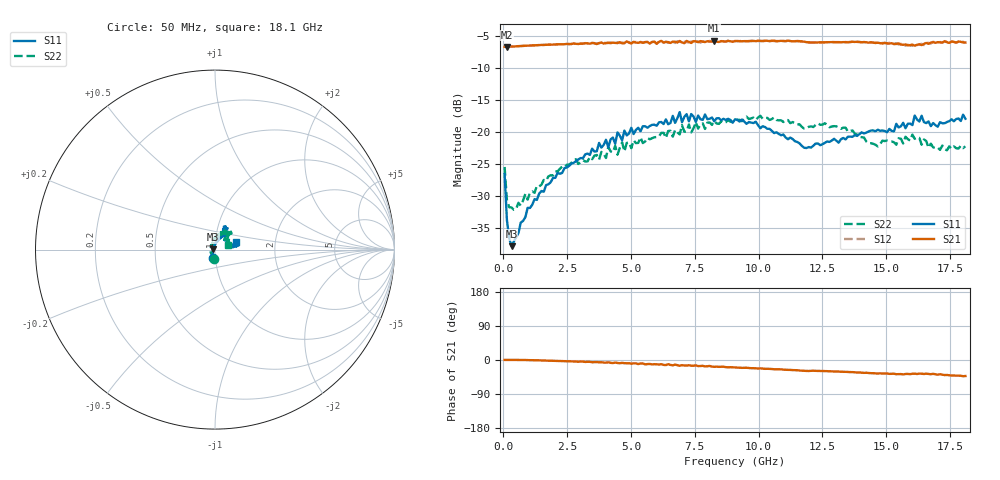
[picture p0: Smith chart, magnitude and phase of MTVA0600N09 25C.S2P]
! Network Analyzer HP8720D.06.14 Serial No. US36140669
!  7 Jul 2005  06:27:09
! Frequency  S11  S21  S12  S22
# HZ  S  DB R 50
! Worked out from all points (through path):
!   201 points, 50 MHz to 18.1 GHz, reference 50 ohm
!   highest |S21| = -5.68 dB at 8.263 GHz (marker M1); lowest = -6.7 dB at 140.2 MHz (marker M2)
!   group delay of S21, straight-line fit = 6.97 ps
!   lowest |S11| = -37.9 dB at 320.8 MHz (marker M3), VSWR 1.03, Z = 48.7 + j0.0733 ohm
!   |S11| at or under -10 dB: start of sweep to end of sweep
!   |S22| runs from -32.2 to -17.5 dB; largest |S21 - S12| = 0.019
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5e7  -26.57 -102.2  -6.65 0.3  -6.68 0.4  -25.48 -94.9
1.4025e8  -33.81 -127.1  -6.69 0.3  -6.68 0.3  -30.67 -144.8
3.2075e8  -37.89 176.6  -6.60 0.5  -6.63 0.5  -31.83 177.1
1.22325e9  -30.52 95.2  -6.43 -0.6  -6.45 -0.6  -29.54 115.1
3.1185e9  -24.10 70.9  -6.16 -4.2  -6.20 -4.5  -24.40 93.6
4.382e9  -21.86 64.8  -6.05 -6.7  -6.05 -7.9  -22.16 85.1
4.47225e9  -20.07 61.2  -6.08 -7.8  -5.97 -7.1  -23.56 87.4
4.65275e9  -21.30 61.3  -6.11 -7.5  -5.98 -8.5  -21.61 86.3
4.743e9  -19.79 64.6  -6.10 -8.4  -6.04 -7.8  -23.05 81.9
6.09675e9  -18.50 63.1  -5.89 -12.0  -5.81 -11.9  -20.72 71.2
6.7285e9  -18.57 67.7  -5.87 -12.1  -6.06 -12.6  -19.69 63.7
6.909e9  -16.89 66.0  -5.75 -15.1  -5.83 -13.8  -20.38 61.6
6.99925e9  -18.48 65.4  -5.97 -13.6  -6.09 -14.9  -18.93 63.2
7.36025e9  -17.19 59.2  -6.05 -15.2  -5.83 -14.6  -20.07 66.2
8.26275e9  -18.34 64.4  -5.68 -18.0  -5.83 -18.4  -18.30 52.9
9.075e9  -18.02 63.3  -5.77 -19.6  -5.74 -19.6  -18.16 50.9
1.21435e10  -22.16 44.6  -5.99 -28.4  -5.95 -28.6  -19.23 52.8
1.512175e10  -19.52 9.6  -6.16 -36.6  -6.03 -36.4  -21.47 41.8
1.602425e10  -18.92 14.4  -6.32 -36.3  -6.51 -37.5  -20.41 35.3
1.61145e10  -17.43 13.7  -6.48 -36.0  -6.23 -36.6  -21.09 35.9
1.7017e10  -19.17 14.3  -5.93 -38.8  -6.05 -39.4  -22.45 28.2
1.81e10  -17.93 20.2  -5.99 -42.3  -6.07 -42.6  -22.24 18.5
